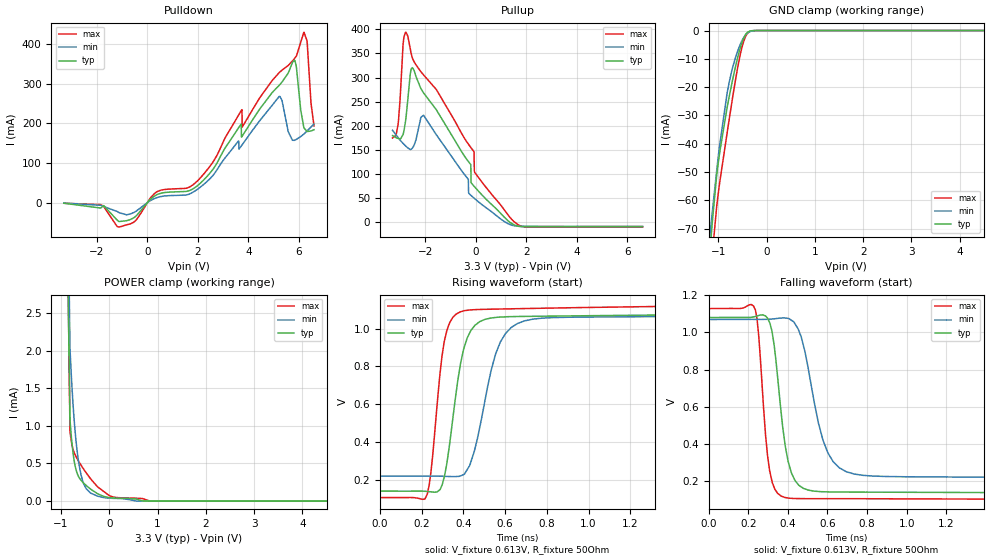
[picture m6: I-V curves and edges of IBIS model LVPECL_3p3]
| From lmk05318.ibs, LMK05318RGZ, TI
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|   LVPECL_3p3 Model
[Model]   LVPECL_3p3
Model_type   3-state
Polarity   Non-Inverting
Vmeas = 0.613
Vref = 0.613
Cref = 2pF
Rref = 50
|   typ   min   max
C_comp   1.41794E-12   1.36037E-12   1.45091E-12
| Where nom  PVT is Nominal Process, 3.3V, 27C
|   Fast PVT is Strong Process,  3.45V, -40C
|   Slow PVT is Weak Process,   3.15V, 125C
[Voltage Range]   3.3   3.15   3.45
|Junction Temperature
[Temperature Range]   27   125   -40
[Pullup Reference]   3.3   3.15   3.45
[Pulldown Reference]   -0   -0   0
[Power Clamp Reference]   3.3   3.15   3.45
[GND Clamp Reference]   0   0   0
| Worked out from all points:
|   slope of the pulldown table from 0 to 0.495 V, typ, clamps not added: 21.6 ohm
|   slope of the pullup table from 0 to 0.495 V, typ, clamps not added: 18.2 ohm
|   GND clamp passes 1 mA (typ) near -0.41 V on its own axis
|   POWER clamp passes 1 mA (typ) near -0.80 V on its own axis
|   falling waveform, V_fixture 0.613V, R_fixture 50Ohm: 20-80 % time 62.7ps typ, 103ps min, 44.4ps max; typ from 1.08 V to 0.138 V
|   rising waveform, V_fixture 0.613V, R_fixture 50Ohm: 20-80 % time 75.2ps typ, 106ps min, 56.1ps max; typ from 0.139 V to 1.08 V
[Pulldown]
|   Voltage   I(typ)   I(min)   I(max)
-3.3V     -1.368mA   -1.115mA   -1.363mA
-1.845V   -13.51mA   -6.485mA   -4.855mA
-1.122V   -47.62mA   -24.89mA   -61.68mA
392.7mV   20.55mA    13.01mA    27.89mA
1.798V    34.42mA    26.05mA    44.53mA
3.739V    166.2mA    144.6mA    233.9mA
5.224V    296.1mA    268.1mA    328.1mA
5.828V    359.1mA    157.3mA    363.5mA
6.204V    188.7mA    173.4mA    429.6mA
6.323V    179.5mA    180.8mA    408.5mA
6.481V    180.8mA    190.7mA    251.3mA
6.6V      184mA      198.2mA    193.6mA
[GND Clamp]
|   Voltage   I(typ)   I(min)   I(max)
-3.3V     -1.225A    -1.029A    -1.515A
-1.181V   -80.15mA   -73.74mA   -92.54mA
-1.132V   -69.26mA   -65.41mA   -80.58mA
-1.122V   -67.19mA   -63.77mA   -78.45mA
-1.033V   -51.11mA   -49.44mA   -62.14mA
-973.5mV  -43.33mA   -40.6mA    -53.92mA
-815.1mV  -26.99mA   -21.86mA   -35.94mA
-765.6mV  -22.62mA   -17.58mA   -30.43mA
-528mV    -5.185mA   -4.26mA    -7.227mA
-438.9mV  -1.534mA   -1.654mA   -2.27mA
-349.8mV  -210.4uA   -427.7uA   -364.9uA
6.6V      0A         0A         0A
[Pullup]
|   Voltage   I(typ)   I(min)   I(max)
-3.3V     179.6mA    190.6mA    174.6mA
-3.082V   173.8mA    175.7mA    202.2mA
-2.884V   181.6mA    163.6mA    367.3mA
-2.765V   217.8mA    157.4mA    393.7mA
-2.498V   319.7mA    154.9mA    338.5mA
-2.072V   268.3mA    221.9mA    305.6mA
-300.3mV  126mA      88.94mA    162.1mA
-280.5mV  124.6mA    59.66mA    160.7mA
-72.6mV   74.57mA    49.88mA    146.1mA
-52.8mV   73.39mA    48.98mA    103.9mA
1.541V    -6.231mA   -7.658mA   -378.7uA
6.6V      -9.523mA   -8.605mA   -10.36mA
[POWER Clamp]
|   Voltage   I(typ)   I(min)   I(max)
-3.3V     2.746A     3.266A     2.249A
-1.488V   31.11mA    34.76mA    35.04mA
-815.1mV  1.082mA    2.027mA    921.9uA
-775.5mV  776.3uA    1.532mA    752.1uA
-726mV    528.1uA    1.059mA    641.3uA
-627mV    314.2uA    482.9uA    520.1uA
-557.7mV  256.3uA    280uA      449.6uA
-478.5mV  207.7uA    164.7uA    374.7uA
-260.7mV  105.7uA    70.86uA    202.7uA
75.9mV    41.45uA    37.03uA    56.03uA
897.6mV   0A         127.3nA    190.2nA
6.6V      0A         0A         0A
[Ramp]
R_load = 50
|   typ   min   max
dV/dt_r   0.5645/7.51806e-11   0.510386/1.05581e-10   0.613931/5.61007e-11
dV/dt_f   0.564762/6.27167e-11   0.50998/1.03357e-10   0.613966/4.44176e-11
[Falling Waveform]
V_fixture = 0.613V
V_fixture_min = 0.648V
V_fixture_max = 0.62V
R_fixture = 50Ohm
C_fixture = 0F
|   Time   V(typ)   V(min)   V(max)
0s        1.08V      1.069V     1.128V
236ps     1.085V     1.07V      1.12V
297.4ps   1.076V     1.07V      338.9mV
330.7ps   932.8mV    1.073V     168.2mV
365.8ps   572.7mV    1.077V     121.7mV
401.1ps   308.6mV    1.075V     111.3mV
455.6ps   179.6mV    1.008V     108.2mV
577.1ps   145mV      422.2mV    107.9mV
694.6ps   143.1mV    252.6mV    107.7mV
2.5ns     138.3mV    218.9mV    104.2mV
[Rising Waveform]
V_fixture = 0.613V
V_fixture_min = 0.648V
V_fixture_max = 0.62V
R_fixture = 50Ohm
C_fixture = 0F
|   Time   V(typ)   V(min)   V(max)
0s        138.5mV    218.3mV    104.2mV
226.8ps   136.8mV    218mV      122.9mV
244.1ps   134.8mV    217.9mV    238.3mV
308.1ps   213.6mV    217.1mV    931mV
384.1ps   800.1mV    218.2mV    1.088V
455.6ps   1.018V     364.6mV    1.1V
532.9ps   1.056V     778.7mV    1.103V
577.1ps   1.061V     928.7mV    1.103V
694.6ps   1.064V     1.041V     1.106V
2.5ns     1.079V     1.069V     1.127V
